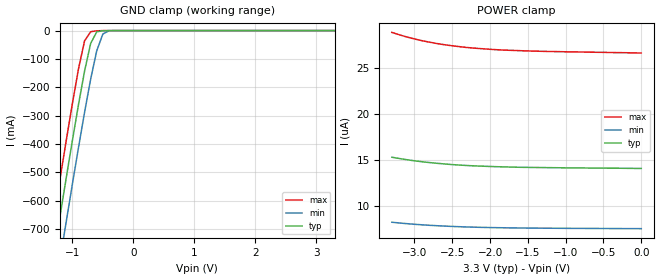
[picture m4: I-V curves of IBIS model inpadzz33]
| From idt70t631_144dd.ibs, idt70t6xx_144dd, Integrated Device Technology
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|   Model inpadzz33
[Model]   inpadzz33
Model_type   Input
Polarity   Non-Inverting
Vinl =  0.80000V
Vinh =  2.00000V
Vmeas =  1.50000V
C_comp   4.50000pF   4.50000pF   4.50000pF
[Temperature Range]   25.00000   100.00000   -40.00000
[Voltage Range]   3.30000V   3.10000V   3.50000V
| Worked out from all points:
|   GND clamp passes 1 mA (typ) near -0.51 V on its own axis
[GND_clamp]
| voltage   I(typ)   I(min)   I(max)
-3.3V     -3.553A    -3.699A    -3.43A
-1.4V     -921.5mA   -1.075A    -790.4mA
-1.3V     -786.2mA   -940.4mA   -654.7mA
-1.2V     -651.9mA   -806.3mA   -520.2mA
-1.1V     -519.1mA   -673.5mA   -387.5mA
-900mV    -262mA     -413.5mA   -136.1mA
-800mV    -143.3mA   -288.9mA   -36.34mA
-700mV    -45.49mA   -171.6mA   -3.982mA
-600mV    -4.315mA   -71.06mA   -846.5uA
-500mV    -419.1uA   -12.18mA   -96.4uA
-400mV    -42.61uA   -832.1uA   -14.65uA
3.3V      14.1uA     7.585uA    26.56uA
[POWER_clamp]
| voltage   I(typ)   I(min)   I(max)
-3.3V     15.31uA    8.274uA    28.82uA
-3.1V     15.04uA    8.118uA    28.32uA
-2.9V     14.82uA    7.993uA    27.92uA
-2.8V     14.73uA    7.941uA    27.76uA
-2.7V     14.65uA    7.895uA    27.61uA
-2.5V     14.51uA    7.818uA    27.37uA
-2.3V     14.41uA    7.759uA    27.18uA
-2.2V     14.37uA    7.736uA    27.11uA
-1.9V     14.28uA    7.683uA    26.94uA
-1.5V     14.21uA    7.642uA    26.81uA
-1V       14.16uA    7.614uA    26.72uA
0V        14.1uA     7.578uA    26.59uA
